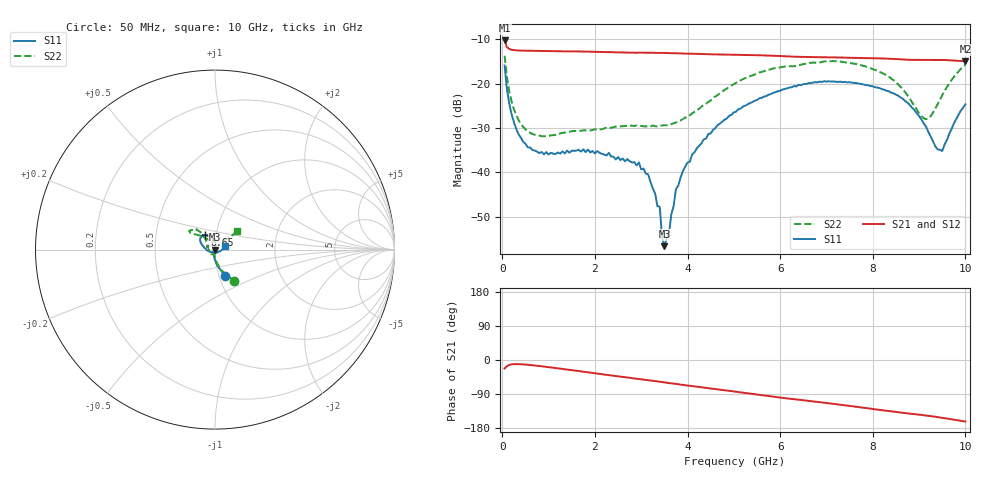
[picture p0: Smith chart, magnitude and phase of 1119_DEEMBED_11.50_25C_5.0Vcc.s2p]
!Hittite Microwave Corp.
!Digital Attenuator/PhaseShifter Rev 1.4.0
!Filename: C:\DATA\DATA\1119_DEEMBED_11.50_25C_5.0Vcc.s2p
!VNA ID: Agilent Technologies,N5224A,MY51441122,A.10.45.03
!Device type:
!2 Port Calibration.
!Temp(C): 25
!Lot Number:
!Serial Number:
!Operator:
!Misc:
!Attenuator:  11.500
# GHZ S DB R 50.0
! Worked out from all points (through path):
!   200 points, 50 MHz to 10 GHz, reference 50 ohm
!   highest |S21| = -10.32 dB at 50 MHz (marker M1); lowest = -15.0 dB at 10 GHz (marker M2)
!   group delay of S21, straight-line fit = 43.2 ps
!   lowest |S11| = -56.6 dB at 3.5 GHz (marker M3), VSWR 1.00, Z = 49.9 - j0.0631 ohm
!   |S11| at or under -10 dB: start of sweep to end of sweep
!   |S22| runs from -31.9 to -13.7 dB; largest |S21 - S12| = 0.0006
!   S11 on the Smith chart (normalised r, x): 50 MHz: 1.07, -0.33; 6.65 GHz: 0.88, +0.15; 10 GHz: 1.12, +0.04
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0.05  -15.93 -69.2  -10.32 -22.2  -10.31 -22.2  -13.75 -58.7
0.1  -21.28 -82.8  -11.81 -16.3  -11.81 -16.3  -18.57 -73.5
0.2  -26.90 -94.6  -12.41 -11.6  -12.41 -11.6  -24.01 -84.3
0.55  -34.35 -115.9  -12.64 -12.6  -12.64 -12.6  -30.71 -95.4
1.75  -34.80 -132.5  -12.81 -30.8  -12.81 -30.9  -30.53 -112.0
2.95  -37.74 -114.6  -13.06 -49.9  -13.07 -50.0  -29.53 -149.0
3.15  -40.43 -109.9  -13.08 -53.2  -13.10 -53.2  -29.59 -158.8
3.4  -47.69 -127.1  -13.11 -57.3  -13.12 -57.4  -29.52 -170.4
3.45  -54.58 -127.5  -13.12 -58.2  -13.13 -58.3  -29.41 -173.2
3.5  -56.56 -154.8  -13.12 -59.0  -13.13 -59.1  -29.39 -176.1
3.6  -53.67 81.3  -13.17 -60.8  -13.18 -60.9  -29.29 178.6
3.75  -43.72 85.6  -13.20 -63.2  -13.20 -63.3  -28.74 170.9
3.95  -38.69 76.6  -13.27 -66.6  -13.28 -66.6  -27.65 159.2
4.45  -31.32 80.8  -13.42 -74.4  -13.43 -74.5  -24.13 138.3
5.05  -26.32 95.0  -13.53 -83.7  -13.55 -83.7  -19.84 128.9
6.65  -19.89 125.1  -14.03 -108.3  -14.04 -108.3  -15.36 139.9
6.7  -19.82 127.0  -14.04 -109.1  -14.06 -109.1  -15.31 140.2
7.65  -19.91 145.5  -14.24 -123.6  -14.25 -123.6  -15.62 145.8
8.35  -21.75 157.4  -14.43 -134.8  -14.43 -134.8  -18.51 137.8
9.15  -29.69 -158.5  -14.68 -146.4  -14.69 -146.5  -28.01 89.1
9.5  -35.15 -65.0  -14.70 -152.6  -14.71 -152.6  -22.59 45.2
10  -24.67 19.7  -15.01 -162.3  -15.01 -162.3  -15.76 40.1
